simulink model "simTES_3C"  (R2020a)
settings: Solver=ode15s  StartTime=0.0  StopTime=tsim  RelTol=1e-3
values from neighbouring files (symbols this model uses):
  dq = 500    [runTES.m]
  dqS = 500    [runTES.m]
  KcEP = 1/kp*1/(tauCEP+thetaEP)    (= 108)    [runTES.m]
  KcSP = 1/kp*1/(tauCSP+thetaSP)    (= 108)    [runTES.m]
  KcTP = 1/kp*1/(tauCTP+thetaTP)    (= 108)    [runTES.m]
  nd = 1    [runTES.m]    (also in Main.m = size(d0,2); Main_OL.m = size(d0,2); runTestCalcBlk.m = size(d0,2); runTransf.m = size(d0,2))
  np = length(param)    [runTES.m]    (also in runH2Psim.m; Main.m = size(p,2); Main_OL.m = size(p,2); runTestCalcBlk.m = size(p,2))
  nu = 4    [runTES.m]    (also in runH2Psim.m = length(u0); Main.m = 1; Main_OL.m = 1; runTestCalcBlk.m = 1)
  nx = 2    [runTES.m]    (also in H2P_Turbine_driven.m = param(end); runTD.m = length(x0); H2P_Boiler_driven.m = param(end); runBD.m = length(x0))
  param = [V;rho;p0;m0;eps]    [runTES.m]    (also in runTD.m = [Tref;TrefB;dHvap;cpg;cpW;cpSt;R;Mwt;     T0;TG0;ME;pC;     ; runBD.m = [Tref;TrefB;dHvap;cpg;cpW;cpSt;R;Mwt;          T0;TG0;ME;pC;; runFP.m = [Tref;TrefB;dHvap;cpg;cpW;cpSt;R;Mwt;          T0;TG0;ME;pC;; runFPV2.m = [Tref;TrefB;dHvap;cpg;cpW;cpSt;R;Mwt;          T0;TG0;ME;pC;)
  pEPs = pTPs - 0.5    (= 4)    [runTES.m]
  ps = p0    (= 5)    [runTES.m]
  pTPs = ps - 0.5    (= 4.5)    [runTES.m]
  qmax = 1000    [runTES.m]
  qS0 = qnom    (= 500)    [runTES.m]
  qsp = qnom    (= 500)    [runTES.m]
  qSP0 = qnom    (= 500)    [runTES.m]
  tauIEP = 4*(tauCEP+thetaEP)    (= 0.0111111111111)    [runTES.m]
  tauISP = 4*(tauCSP+thetaSP)    (= 0.0111111111111)    [runTES.m]
  tauITP = 4*(tauCTP+thetaTP)    (= 0.0111111111111)    [runTES.m]
  tauTEP = tauIEP/2    (= 0.00555555555556)    [runTES.m]
  tauTSP = tauISP/2    (= 0.00555555555556)    [runTES.m]
  tauTTP = tauITP/2    (= 0.00555555555556)    [runTES.m]
  td1 = 1    [runTES.m]
  td2 = 15    [runTES.m]
  tq1 = 12    [runTES.m]
  tq2 = 40    [runTES.m]
  Vmax = V    (= 5000)    [runTES.m]
  x0 = [Vh0;p0]    [runTES.m]    (also in runTD.m = [TE0;TD0;TSh0;MD0; MSh0;w0;TA0;0;0;0;0;0;0;0;0;0]; runBD.m = [TE0;TD0;TSh0;MD0; MSh0;w0;TA0;0;0;0;0;0;0;0;0;0]; runFP.m = [TE0;TD0;TSh0;MD0; MSh0;w0;TA0;0;0;0;0;0;0;0]; runFPV2.m = [TE0;TD0;TSh0;MD0; MSh0;w0;TA0;0;0;0;0;0;0;0])
undefined symbols (not defined in the file or in its folder): ChargingPolicy, DischargingPolicy, TESmodel

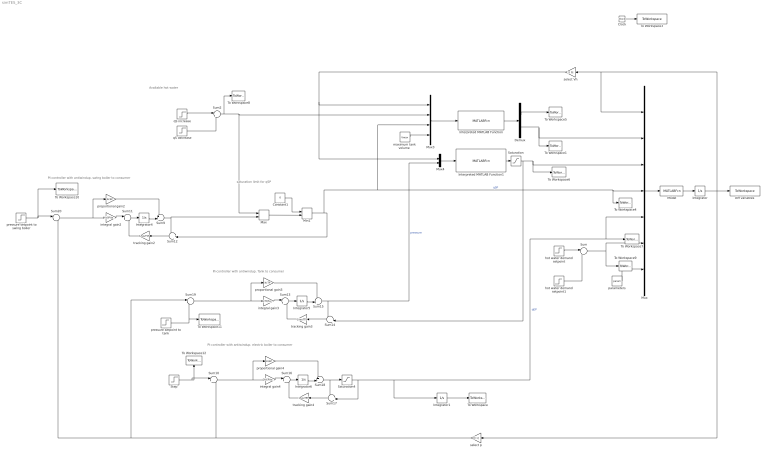
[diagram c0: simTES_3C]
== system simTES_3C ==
  note: saturation limit for qSP
  note: PI-controller with antiwindup. swing boiler to consumer
  note: PI-controller with antiwindup. Tank to consumer
  note: PI-controller with antiwindup. electric boiler to consumer
  note: Available hot water
  Clock : Clock
  Constant1 : Constant  Value=0
  Demux : Demux  Outputs=2
  Integrator : Integrator  InitialCondition=x0
  Integrator1 : Integrator
  Integrator4 : Integrator  InitialCondition=qSP0
  Integrator5 : Integrator
  Integrator6 : Integrator
  Interpreted MATLAB Function : MATLABFcn  MATLABFcn=ChargingPolicy(u(1),u(2),u(3),u(4))  OutputDimensions=2
  Interpreted MATLAB Function1 : MATLABFcn  MATLABFcn=DischargingPolicy(u(1),u(2))  OutputDimensions=1
  Max : MinMax  Inputs=2  ZeroCross=off
  Min1 : MinMax  Function=max  Inputs=2  ZeroCross=off
  Model : MATLABFcn  MATLABFcn=TESmodel(u(1:nx),u(nx+1:nx+nu),u(nx+nu+1:nx+nu+nd),u(nx+nu+nd+1:nx+nu+nd+np))  OutputDimensions=nx
  Mux : Mux  Inputs=7
  Mux3 : Mux
  Mux4 : Mux  Inputs=2
  Saturation : Saturate  UpperLimit=qmax  LowerLimit=0  ZeroCross=off
  Saturation4 : Saturate  UpperLimit=qmax  LowerLimit=0
  Step : Step  Before=pEPs  After=pEPs  SampleTime=0  ZeroCross=off
  Sum : Sum  Inputs=|+-
  Sum10 : Sum  Inputs=|+-
  Sum{2,11,13,16} (4 alike) : Sum  Inputs=|++
  Sum12 : Sum  Inputs=-+|
  Sum14 : Sum  Inputs=-+|
  Sum15 : Sum  Inputs=++|
  Sum17 : Sum  Inputs=-+|
  Sum18 : Sum  Inputs=++|
  Sum19 : Sum  Inputs=|-+
  Sum20 : Sum  Inputs=|+-
  Sum9 : Sum  Inputs=++|
  To Workspace : ToWorkspace  VariableName=J3C  SampleTime=-1
  To Workspace1 : ToWorkspace  VariableName=qST3C  SampleTime=-1
  To Workspace10 : ToWorkspace  VariableName=pref  SampleTime=-1
  To Workspace11 : ToWorkspace  VariableName=pTPref  SampleTime=-1
  To Workspace12 : ToWorkspace  VariableName=pEPref  SampleTime=-1
  To Workspace3 : ToWorkspace  VariableName=t3C  SampleTime=-1
  To Workspace4 : ToWorkspace  VariableName=qSP3C  SampleTime=-1
  To Workspace5 : ToWorkspace  VariableName=qD3C  SampleTime=-1
  To Workspace6 : ToWorkspace  VariableName=qTP3C  SampleTime=-1
  To Workspace7 : ToWorkspace  VariableName=qEP3C  SampleTime=-1
  To Workspace8 : ToWorkspace  VariableName=qS  SampleTime=-1
  To Workspace9 : ToWorkspace  VariableName=qref  SampleTime=-1
  diff variables : ToWorkspace  VariableName=y3C  SampleTime=-1
  hot water demand setpoint : Step  Time=tq1  Before=qsp  After=qsp+dq  SampleTime=0  ZeroCross=off
  hot water demand setpoint1 : Step  Time=tq2  After=dq*1.5  SampleTime=0
  integral gain2 : Gain  Gain=KcSP/tauISP  Multiplication=Matrix(K*u)
  integral gain3 : Gain  Gain=KcTP/tauITP  Multiplication=Matrix(K*u)
  integral gain4 : Gain  Gain=KcEP/tauIEP  Multiplication=Matrix(K*u)
  "maximum tank volume " : Constant  Value=Vmax
  parameters : Constant  Value=param
  pressure setpoint to swing boiler : Step  Before=ps  After=ps  SampleTime=0  ZeroCross=off
  pressure setpoint to tank : Step  Before=pTPs  After=pTPs  SampleTime=0  ZeroCross=off
  proportional gain2 : Gain  Gain=KcSP  Multiplication=Matrix(K*u)
  proportional gain3 : Gain  Gain=KcTP  Multiplication=Matrix(K*u)
  proportional gain4 : Gain  Gain=KcEP  Multiplication=Matrix(K*u)
  qS decrease : Step  Time=td2  After=-dqS  SampleTime=0  ZeroCross=off
  qS increase : Step  Time=td1  Before=qS0  After=qS0+dqS  SampleTime=0  ZeroCross=off
  select Vh : Gain  Gain=[1 0]  Multiplication=Matrix(K*u)
  select p : Gain  Gain=[0 1]  Multiplication=Matrix(K*u)
  tracking gain2 : Gain  Gain=1/tauTSP  Multiplication=Matrix(K*u)
  tracking gain3 : Gain  Gain=1/tauTTP  Multiplication=Matrix(K*u)
  tracking gain4 : Gain  Gain=1/tauTEP  Multiplication=Matrix(K*u)
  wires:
  Step/1 -> Sum10/1, To Workspace12/1
  Sum11/1 -> Integrator4/1
  Sum9/1 -> Sum12/1, Max/2
  Sum12/1 -> tracking gain2/1
  tracking gain2/1 -> Sum11/2
  Min1/1 -> Mux3/3, To Workspace4/1, Mux/4, Sum12/2  "qSP"
  Integrator4/1 -> Sum9/2
  integral gain2/1 -> Sum11/1
  proportional gain2/1 -> Sum9/1
  proportional gain3/1 -> Sum15/1
  integral gain3/1 -> Sum13/1
  Sum19/1 -> proportional gain3/1, integral gain3/1
  Integrator5/1 -> Sum15/2
  tracking gain3/1 -> Sum13/2
  Sum14/1 -> tracking gain3/1
  Sum13/1 -> Integrator5/1
  Sum15/1 -> Mux4/2, Sum14/1  "pressure"
  proportional gain4/1 -> Sum18/1
  integral gain4/1 -> Sum16/1
  Sum10/1 -> proportional gain4/1, integral gain4/1
  Integrator6/1 -> Sum18/2
  tracking gain4/1 -> Sum16/2
  Sum17/1 -> tracking gain4/1
  Sum18/1 -> Saturation4/1, Sum17/1
  Sum16/1 -> Integrator6/1
  Saturation4/1 -> Integrator1/1, To Workspace7/1, Mux/5, Sum17/2  "qEP"
  pressure setpoint to tank/1 -> Sum19/2, To Workspace11/1
  Max/1 -> Min1/2
  Constant1/1 -> Min1/1
  Sum20/1 -> proportional gain2/1, integral gain2/1
  Saturation/1 -> To Workspace6/1, Mux/3, Sum14/2
  Mux3/1 -> Interpreted MATLAB Function/1
  "maximum tank volume "/1 -> Mux3/4
  Interpreted MATLAB Function/1 -> Demux/1
  Demux/2 -> To Workspace1/1, Mux/2
  Mux4/1 -> Interpreted MATLAB Function1/1
  Sum/1 -> To Workspace9/1, Mux/6
  Demux/1 -> To Workspace5/1
  parameters/1 -> Mux/7
  qS decrease/1 -> Sum2/2
  Integrator/1 -> Mux/1, select Vh/1, diff variables/1, select p/1
  Sum2/1 -> To Workspace8/1, Mux3/2, Max/1
  qS increase/1 -> Sum2/1
  Model/1 -> Integrator/1
  Clock/1 -> To Workspace3/1
  select Vh/1 -> Mux4/1, Mux3/1
  Mux/1 -> Model/1
  Interpreted MATLAB Function1/1 -> Saturation/1
  select p/1 -> Sum10/2, Sum20/2, Sum19/1
  pressure setpoint to swing boiler/1 -> To Workspace10/1, Sum20/1
  hot water demand setpoint1/1 -> Sum/2
  hot water demand setpoint/1 -> Sum/1
  Integrator1/1 -> To Workspace/1
